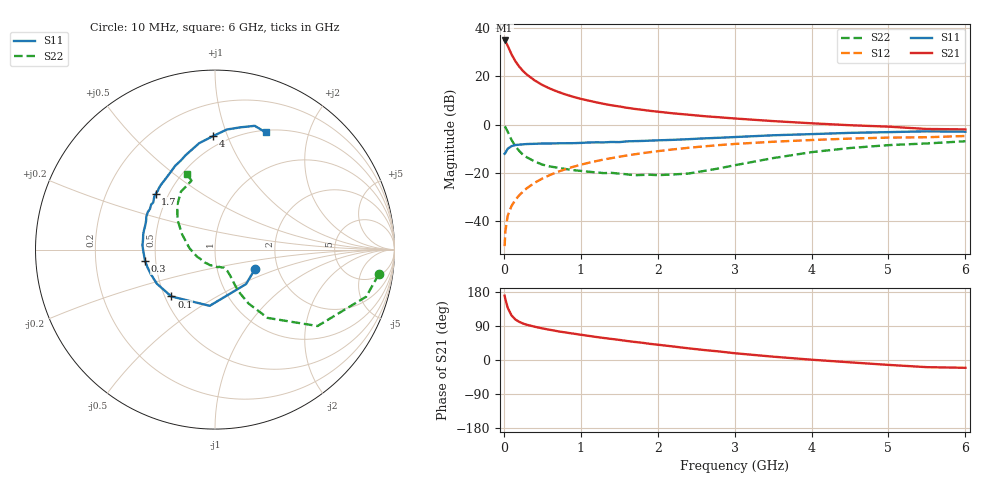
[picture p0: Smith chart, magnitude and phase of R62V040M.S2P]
! SIEMENS Small Signal Semiconductors
! BFR193
! Si NPN RF Bipolar Junction Transistor in SOT23
! VCE = 2 V  IC = 40 mA
! Common Emitter S-Parameters:  May  1996
# GHz  S  MA  R  50
!  f  S11  S21  S12  S22
! GHz  MAG  ANG  MAG  ANG  MAG  ANG  MAG  ANG
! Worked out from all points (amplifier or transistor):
!   36 points, 10 MHz to 6 GHz, reference 50 ohm
!   highest |S21| = 34.9 dB at 10 MHz (marker M1)
!   |S21| within 3 dB of that: start of sweep to 61.34 MHz
!   unconditionally stable (mu >= 1): 399.9 MHz to 1.933 GHz
!   at 250 MHz: K = 0.95, MSG = 25.0 dB, |S12| = -27.8 dB
!   at 1.4 GHz: K = 1.02, MAG = 10.1 dB, |S12| = -13.9 dB
!   at 6 GHz: K = 0.96, MSG = 1.4 dB, |S12| = -4.7 dB
!   S11 on the Smith chart (normalised r, x): 10 MHz: 1.53, -0.35; 100 MHz: 0.54, -0.32; 300 MHz: 0.44, -0.07; 1.7 GHz: 0.43, +0.33; 4 GHz: 0.42, +0.89; 6 GHz: 0.52, +1.39
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0.01  0.248 -25.9  55.59 169.8  0.003 82.8  0.9226 -8.6
0.02  0.2584 -48.0  53.6 160.2  0.0061 78.2  0.8822 -17.3
0.05  0.3147 -95.4  43.19 138.0  0.0128 70.0  0.7126 -36.7
0.1  0.3568 -133.0  28.67 117.6  0.0205 68.3  0.4804 -52.4
0.15  0.3756 -149.6  20.6 106.9  0.0274 69.1  0.3537 -58.1
0.2  0.3833 -159.4  15.95 100.7  0.0341 70.5  0.2837 -60.1
0.25  0.3892 -165.7  12.89 96.2  0.0408 71.7  0.2361 -60.7
0.3  0.3947 -170.8  10.86 92.9  0.0479 72.7  0.209 -60.4
0.4  0.399 -178.1  8.272 87.9  0.0619 73.9  0.1719 -59.8
0.5  0.4048 176.7  6.63 83.4  0.0758 73.6  0.1477 -59.8
0.6  0.4048 172.2  5.57 79.7  0.09 72.8  0.135 -60.2
0.7  0.4087 168.2  4.801 75.9  0.1042 72.0  0.1276 -61.1
0.8  0.4101 164.7  4.22 72.7  0.1183 70.9  0.1199 -62.1
1.1  0.4245 154.4  3.147 63.8  0.1606 67.5  0.1052 -69.9
1.4  0.4356 144.7  2.509 55.6  0.2013 63.0  0.0996 -79.9
1.7  0.4532 136.8  2.115 47.7  0.2415 58.8  0.0888 -96.0
2.2  0.4819 124.6  1.709 35.7  0.3052 51.0  0.0923 -129.6
3.5  0.5993 98.5  1.181 8.8  0.44 30.1  0.2014 155.3
4  0.6338 90.8  1.063 0.8  0.478 23.1  0.2678 141.4
4.5  0.6726 84.3  0.969 -6.2  0.5118 16.0  0.3262 130.1
5.5  0.7243 72.2  0.81 -18.9  0.5455 2.1  0.4058 108.8
6  0.7116 66.7  0.794 -20.6  0.5796 -1.9  0.4504 110.6
